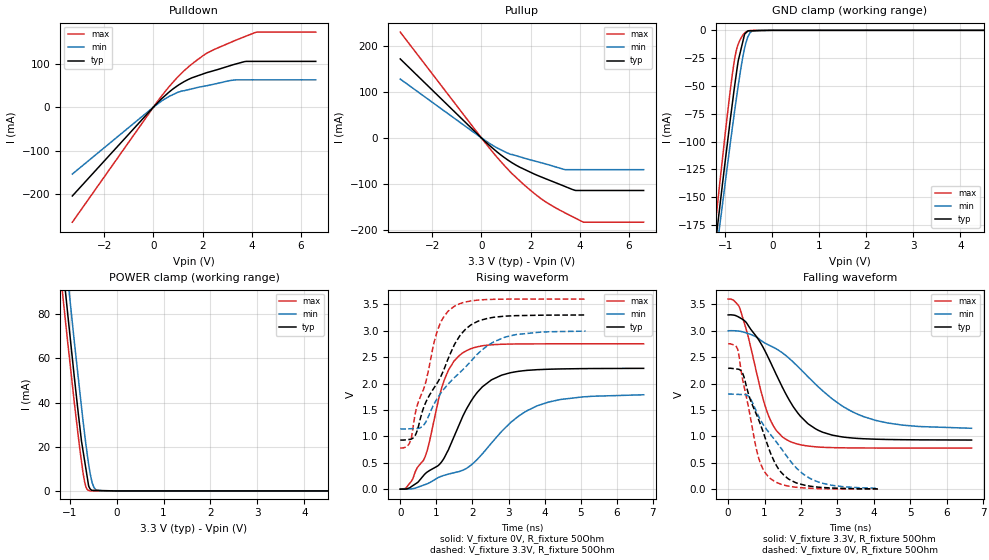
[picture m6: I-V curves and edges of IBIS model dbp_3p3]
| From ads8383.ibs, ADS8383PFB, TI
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|   dbp_3p3 Model
[Model]   dbp_3p3
Model_type   3-state
Polarity   Non-Inverting
Vmeas = 1.65
Vref = 1.65
Cref = 10pF
Rref = 50
|   typ   min   max
|   (nom PVT)   (fast PVT)   (slow PVT)
|C_comp from frequency sweep method (F=250KHz)
|C_comp   1.832e-11   1.472e-11   2.111e-11
|ON state : BUFFER OUTPUT TURNED HIGH
|C_comp   1.832e-11   1.472e-11   2.111e-11
|OFF state: BUFFER IN HIGH IMPEDANCE
|C_comp   2.315e-11   2.198e-11   2.424e-11
|C_comp from LC tank measurement(L=1nH)
|Resonant Frequency(Hz)   2.070e+09   2.200e+09   1.970e+09
C_comp   5.917e-12   5.239e-12   6.533e-12
|ON state : BUFFER OUTPUT TURNED HIGH
|Resonant Frequency(Hz)   2.070e+09   2.200e+09   1.970e+09
|C_comp   5.917e-12   5.239e-12   6.533e-12
|OFF state: BUFFER IN HIGH IMPEDANCE
|Resonant Frequency(Hz)   1.940e+09   1.960e+09   1.930e+09
|C_comp   6.737e-12   6.600e-12   6.807e-12
| Where nom  PVT is Nominal Process, 3.3V, 35C
|   Fast PVT is Strong Process,  3.6V, -40C
|   Slow PVT is Weak Process,   3V, 95C
[Voltage Range]   3.3   3   3.6
|Ambient Temperature   25   85   -40
|Junction Temperature
[Temperature Range]   35   95   -40
[Pullup Reference]   3.3   3   3.6
[Pulldown Reference]   0   0   0
[Power Clamp Reference]   3.3   3   3.6
[GND Clamp Reference]   0   0   0
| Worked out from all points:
|   slope of the pulldown table from 0 to 0.495 V, typ, clamps not added: 18 ohm
|   slope of the pullup table from 0 to 0.495 V, typ, clamps not added: 20.6 ohm
|   GND clamp passes 1 mA (typ) near -0.53 V on its own axis
|   POWER clamp passes 1 mA (typ) near -0.56 V on its own axis
|   falling waveform, V_fixture 3.3V, R_fixture 50Ohm: 20-80 % time 1.12ns typ, 1.88ns min, 646ps max; typ from 3.3 V to 0.931 V
|   rising waveform, V_fixture 0V, R_fixture 50Ohm: 20-80 % time 1.06ns typ, 1.66ns min, 657ps max; typ from 0 V to 2.29 V
|   rising waveform, V_fixture 3.3V, R_fixture 50Ohm: 20-80 % time 993ps typ, 1.38ns min, 656ps max; typ from 0.93 V to 3.3 V
|   falling waveform, V_fixture 0V, R_fixture 50Ohm: 20-80 % time 767ps typ, 1.12ns min, 491ps max; typ from 2.29 V to 0.007 V
[Pulldown]
|   Voltage   I(typ)   I(min)   I(max)
-3.3V     -204.6mA   -154.2mA   -265mA
18mV      1.08mA     836.9uA    1.444mA
326.7mV   19.01mA    13.8mA     25.15mA
633mV     34.53mA    24.58mA    46.83mA
1.092V    53.49mA    35.65mA    75.18mA
1.706V    70.25mA    44.03mA    105.5mA
2.167V    79.35mA    49.27mA    124mA
2.473V    84.25mA    53mA       132.8mA
3.087V    94.87mA    60.87mA    147.7mA
3.703V    104.7mA    62.84mA    162mA
4.162V    105.3mA    62.84mA    172.3mA
6.6V      105.3mA    62.84mA    172.7mA
[GND Clamp]
|   Voltage   I(typ)   I(min)   I(max)
-3.3V     -974.2mA   -933.7mA   -1.034A
-1.314V   -229.7mA   -240.8mA   -214.7mA
-1.191V   -184.5mA   -199.2mA   -165.9mA
-1.127V   -161.4mA   -177.9mA   -140.3mA
-896.4mV  -80.46mA   -101.8mA   -54mA
-806.4mV  -51.03mA   -73.5mA    -26.54mA
-726mV    -27.31mA   -49.54mA   -12.39mA
-590.7mV  -3.416mA   -16mA      -2.461mA
-522mV    -661.5uA   -5.824mA   -511.5uA
-432mV    -420.6uA   -687.9uA   -28.88uA
-285mV    -276.4uA   -8.015uA   -14.67uA
6.6V      0A         0A         0A
[Pullup]
|   Voltage   I(typ)   I(min)   I(max)
-3.3V     171.7mA    128mA      230.1mA
390mV     -19.24mA   -14.1mA    -26.25mA
1.071V    -47.97mA   -33.28mA   -68.01mA
1.247V    -54.19mA   -36.09mA   -77.78mA
2.167V    -79.04mA   -50.28mA   -121.6mA
2.646V    -89.58mA   -57.16mA   -140.4mA
3.393V    -105.5mA   -69.02mA   -162.9mA
3.825V    -114.4mA   -69.13mA   -174.6mA
4.144V    -114.4mA   -69.13mA   -183.2mA
6.6V      -114.4mA   -69.13mA   -183.4mA
[POWER Clamp]
|   Voltage   I(typ)   I(min)   I(max)
-3.3V     570.5mA    585.2mA    553.5mA
-1.197V   113.1mA    129.2mA    99.07mA
-1.044V   81.14mA    97.27mA    68.17mA
-1.033V   78.82mA    95mA       66.02mA
-897.6mV  51.33mA    67.38mA    39.83mA
-720mV    19.09mA    33.02mA    9.234mA
-651.6mV  9.98mA     21.04mA    1.855mA
-594mV    2.312mA    12.14mA    162.5uA
-528mV    273.9uA    4.51mA     21.55uA
-480mV    248.9uA    1.524mA    9.975uA
-285mV    147.1uA    4.123uA    53.13nA
6.6V      0A         0A         0A
[Ramp]
R_load = 50
|   typ   min   max
dV/dt_r   1.37315/1.06235e-09   1.0802/1.66694e-09   1.65133/6.52364e-10
dV/dt_f   1.42183/1.11623e-09   1.11572/1.89406e-09   1.69251/6.4498e-10
[Falling Waveform]
V_fixture = 3.3V
V_fixture_min = 3V
V_fixture_max = 3.6V
R_fixture = 50Ohm
|   Time   V(typ)   V(min)   V(max)
0s        3.3V       3V         3.6V
322ps     3.246V     2.991V     3.422V
1.058ns   2.553V     2.749V     1.485V
1.31ns    2.186V     2.662V     1.124V
1.568ns   1.824V     2.54V      952.8mV
1.984ns   1.382V     2.274V     841.1mV
2.398ns   1.144V     1.988V     803.1mV
3.706ns   956mV      1.377V     780.9mV
4.786ns   937.4mV    1.214V     779.4mV
6.682ns   931.4mV    1.154V     779.2mV
[Rising Waveform]
V_fixture = 0V
V_fixture_min = 0V
V_fixture_max = 0V
R_fixture = 50Ohm
|   Time   V(typ)   V(min)   V(max)
0s        6.807nV    15.05nV    5.351nV
302ps     44.89mV    5.094mV    142.8mV
686ps     288.6mV    86.07mV    608.4mV
1.218ns   591.7mV    262mV      2.063V
1.736ns   1.385V     359.9mV    2.584V
2.112ns   1.814V     549.6mV    2.691V
2.524ns   2.068V     870.5mV    2.734V
3.078ns   2.208V     1.273V     2.748V
3.78ns    2.262V     1.574V     2.752V
6.744ns   2.288V     1.787V     2.752V
[Rising Waveform]
V_fixture = 3.3V
V_fixture_min = 3V
V_fixture_max = 3.6V
R_fixture = 50Ohm
|   Time   V(typ)   V(min)   V(max)
0s        930.1mV    1.14V      779mV
252ps     941.8mV    1.143V     864.4mV
416ps     1.02V      1.147V     1.434V
670ps     1.584V     1.231V     1.942V
1.032ns   2.019V     1.728V     3.004V
1.386ns   2.564V     2.033V     3.404V
1.748ns   2.984V     2.272V     3.534V
2.216ns   3.197V     2.606V     3.584V
3.204ns   3.286V     2.927V     3.599V
5.134ns   3.299V     2.993V     3.6V
[Falling Waveform]
V_fixture = 0V
V_fixture_min = 0V
V_fixture_max = 0V
R_fixture = 50Ohm
|   Time   V(typ)   V(min)   V(max)
0s        2.289V     1.801V     2.752V
262ps     2.275V     1.796V     2.647V
406ps     2.181V     1.794V     2.047V
556ps     1.807V     1.762V     1.561V
806ps     1.367V     1.424V     669.5mV
966ps     1.073V     1.221V     367.9mV
1.13ns    744.6mV    1.064V     219.4mV
1.528ns   267.2mV    703.1mV    78.29mV
2.27ns    54.8mV     195.3mV    16.93mV
4.108ns   6.794mV    17.63mV    1.151mV
